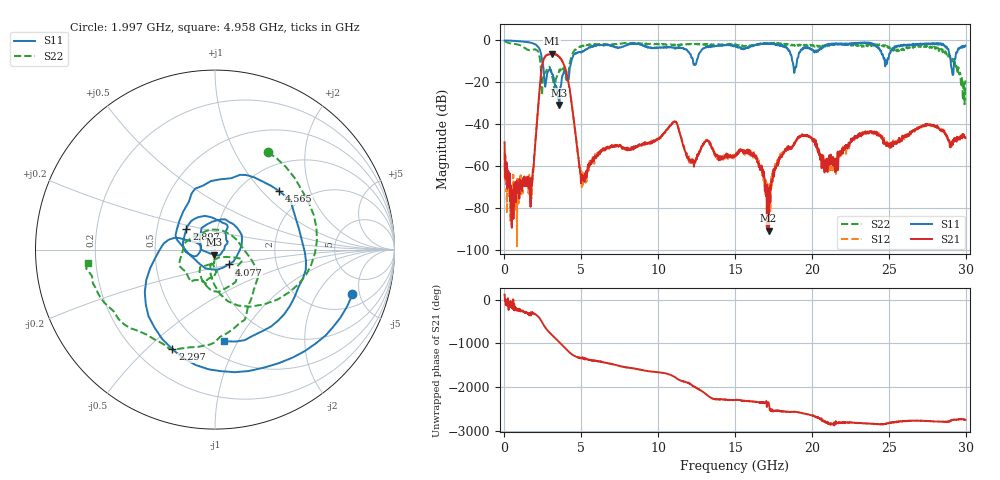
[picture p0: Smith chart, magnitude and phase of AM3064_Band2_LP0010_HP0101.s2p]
# Hz S DB R 50.0
!freq dBS11 angS11 dBS21 angS21 dBS12 angS12 dBS22 angS22
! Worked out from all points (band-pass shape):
!   1600 points, 10 MHz to 29.98 GHz, reference 50 ohm
!   highest |S21| = -6.38 dB at 3.084 GHz (marker M1); lowest = -90.9 dB at 17.18 GHz (marker M2)
!   |S21| within 3 dB of the highest: 2.54 GHz to 3.716 GHz (1.176 GHz wide, 37.6 % of centre)
!   lowest |S11| = -30.9 dB at 3.571 GHz (marker M3), VSWR 1.06, Z = 49.2 - j2.71 ohm
!   |S11| at or under -10 dB: 2.46 GHz to 4.347 GHz (1.887 GHz wide, 55.4 % of centre); 18.73 GHz to 19.02 GHz (290.4 MHz wide, 1.54 % of centre); 29.02 GHz to 29.25 GHz (229.2 MHz wide, 0.786 % of centre)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
!   |S22| runs from -30.6 to -0.2 dB; largest |S21 - S12| = 0.015
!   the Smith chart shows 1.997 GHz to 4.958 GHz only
!   S11 on the Smith chart (normalised r, x): 1.997 GHz: 3.00, -4.26; 2.297 GHz: 0.35, -0.60; 2.897 GHz: 0.71, +0.17; 4.077 GHz: 1.15, -0.19; 4.565 GHz: 1.48, +1.26; 4.958 GHz: 0.63, -0.88
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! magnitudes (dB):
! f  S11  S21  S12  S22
! 10 MHz  0.0  -48.6  -53.5  -0.2
! 516.1 MHz  -0.2  -75.9  -71.8  -1.5
! 1.716 GHz  -1.1  -65.8  -75.5  -4.6
! 1.997 GHz  -1.9  -50.1  -49.9  -4.2
! 2.297 GHz  -4.4  -22.5  -22.5  -8.5
! 2.897 GHz  -14.2  -6.7  -6.6  -12.6
! 3.084 GHz  -15.8  -6.4  -6.4  -16.6
! 3.571 GHz  -30.9  -7.9  -7.9  -14.0
! 4.077 GHz  -18.9  -17.0  -16.9  -18.9
! 4.565 GHz  -6.3  -41.3  -41.3  -4.5
! 4.958 GHz  -5.8  -64.8  -63.3  -2.9
! 5.015 GHz  -5.7  -64.1  -66.6  -2.9
! 10 GHz  -3.5  -47.2  -46.9  -1.8
! 15 GHz  -2.6  -54.9  -55.8  -1.9
! 16.28 GHz  -2.2  -55.9  -54.5  -2.2
! 17.18 GHz  -1.8  -90.9  -77.4  -1.5
! 18.02 GHz  -2.6  -55.9  -53.8  -1.8
! 19.99 GHz  -4.2  -47.3  -46.8  -2.2
! 20.87 GHz  -2.2  -57.1  -57.3  -2.9
! 25 GHz  -8.2  -50.0  -49.9  -2.9
! 28.56 GHz  -2.3  -43.0  -42.9  -4.7
! 29.98 GHz  -2.5  -46.7  -46.0  -19.2
